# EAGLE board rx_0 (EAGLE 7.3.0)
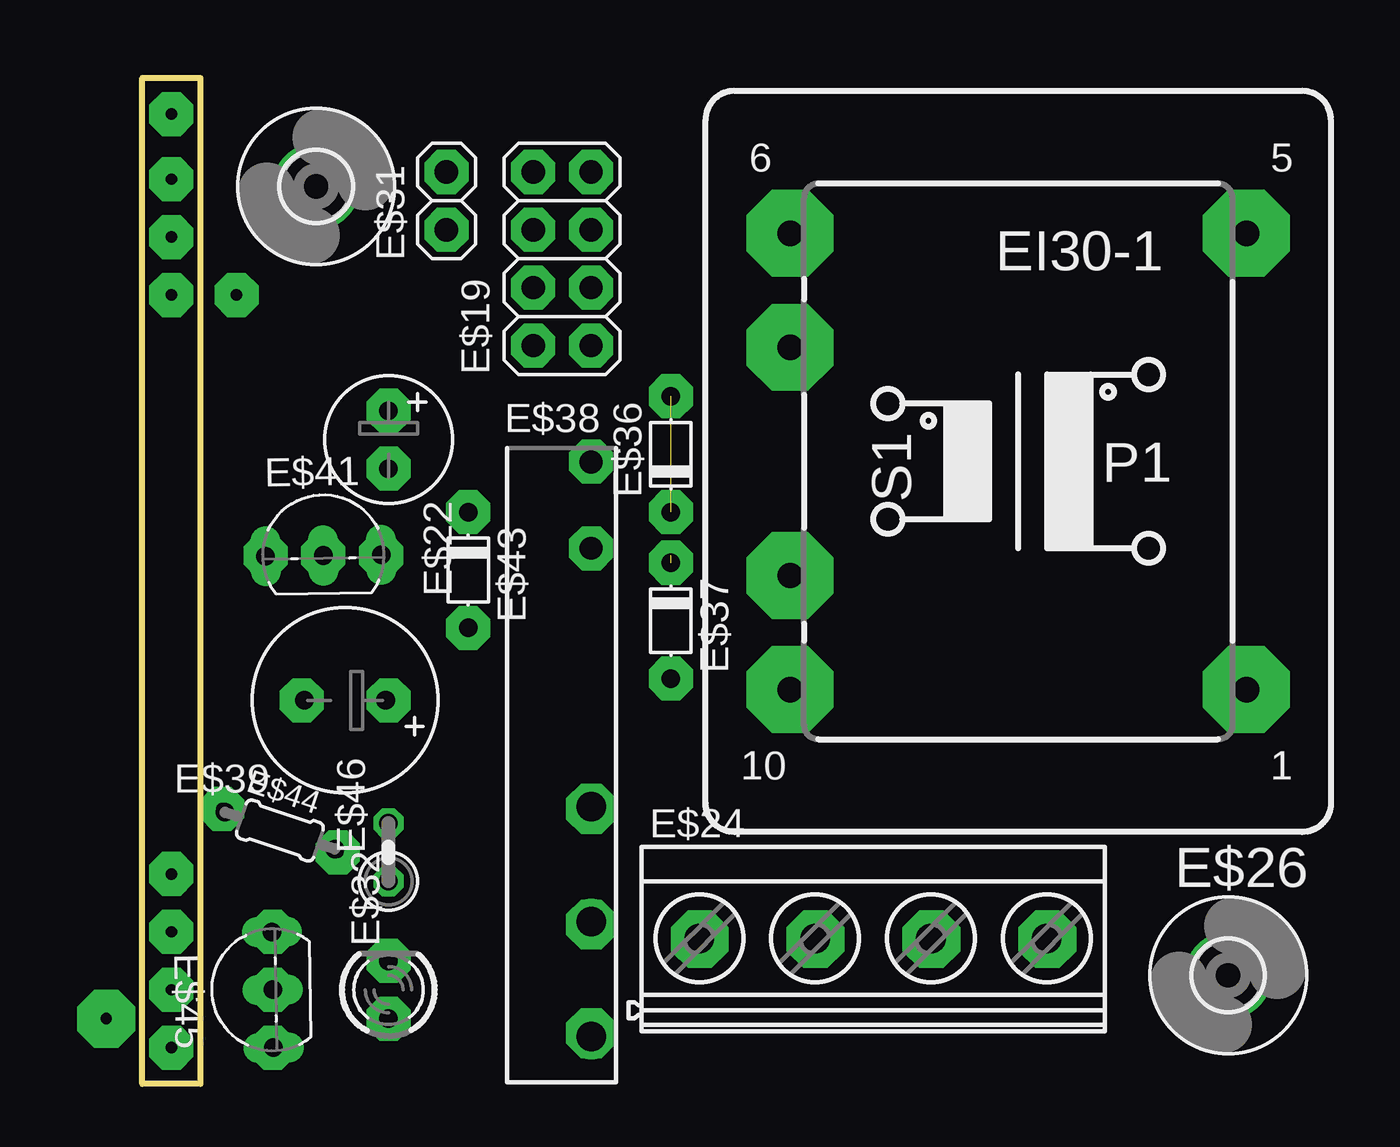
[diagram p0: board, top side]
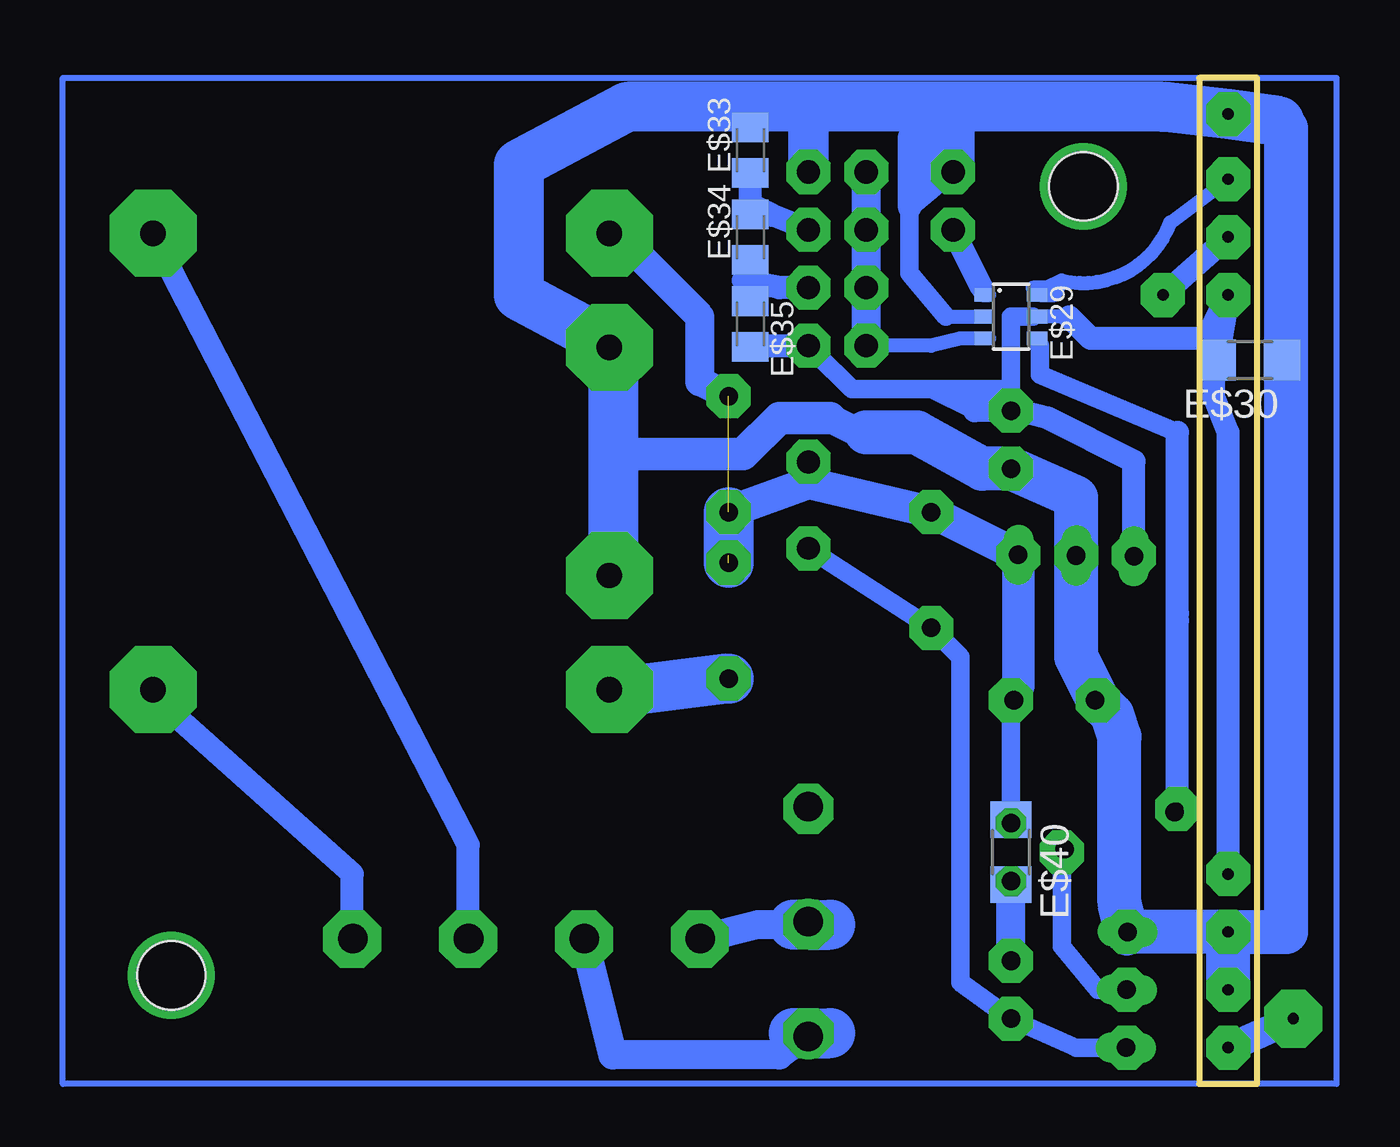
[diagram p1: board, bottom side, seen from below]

Size 2.54 x 44.13 mm. Coordinates in mm from the lower left corner, seen from the top.
Outline: 0,44.13 2.54,44.13 2.54,0 0,0 0,44.13
Copper layers (1*16): Top 0.035mm / dielectric 1.5mm / Bottom 0.035mm
Design rules "default": minimum track width 10mil, minimum drill 24mil, track to track 8mil, track to pad 8mil, pad to pad 8mil, via to via 8mil, smd to smd 8mil, copper to edge 40mil, drill to drill 8mil, minimum pad ring 10mil, minimum via ring 8mil, stop-mask expansion 4mil, vias tented up to drill 0mil, thermal gap 10mil

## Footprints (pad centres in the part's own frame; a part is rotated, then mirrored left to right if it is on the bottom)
2X04 = drill 1.016 octagon: 1 -3.81,-1.27; 2 -3.81,1.27; 3 -1.27,-1.27; 4 -1.27,1.27; 5 1.27,-1.27; 6 1.27,1.27; 7 3.81,-1.27; 8 3.81,1.27
E2,5-6 = drill 0.813 pad 1.6: + -1.27,0 | drill 0.813 pad 1.6 octagon: - 1.27,0
MKDSN1,5/4-5,08 = drill 1.3 pad 2: 1 -7.641,0.025; 2 -2.561,0.025; 3 2.519,0.025; 4 7.599,0.025
EI30-1 = drill 1.118 pad 3.81 octagon: 1 -10.008,10.008; 5 -10.008,-10.008; 6 10.008,-10.008; 7 10.008,-5.004; 9 10.008,5.004; 10 10.008,10.008
3,0 = hole 3: 0,0
SOT23-6 = smd 0.6 x 0.9: 1 -0.95,-1.15; 2 0,-1.15; 3 0.95,-1.15; 4 0.95,1.15; 5 0,1.15; 6 -0.95,1.15
R1206 = smd 1.6 x 1.803: 1 -1.422,0; 2 1.422,0
1X02 = drill 1.016 octagon: 1 -1.27,0; 2 1.27,0
LED3MM = drill 0.813 octagon: A -1.27,0; K 1.27,0
C0805K = smd 1.3 x 1.6: 1 -1,0; 2 1,0
D-5 = drill 0.813 octagon: A 2.54,0; C -2.54,0
FTR-LYC = drill 1 pad 1.6: 1 -3.78,0; 2 0,0 | drill 1.3 pad 2: 3 11.34,0; 4 16.38,0; 5 21.42,0
E3,5-8 = drill 0.813 pad 1.6: + -1.778,0 | drill 0.813 pad 1.6 octagon: - 1.778,0
TO92-BCE = drill 0.813 long: B 2.54,0; C 0,0; E -2.54,0
0204/5 = drill 0.813 octagon: 1 -2.54,0; 2 2.54,0
0207/2V = drill 0.813 octagon: 1 -1.27,0; 2 1.27,0

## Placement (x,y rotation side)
E$19  [2X04]  18.41,36.2 90 top  (outside the outline)
E$22  [E2,5-6]  not placed on the board
E$24  [MKDSN1,5/4-5,08]  not placed on the board
E$26  [EI30-1]  not placed on the board
E$28  [3,0]  not placed on the board
E$29  [SOT23-6]  not placed on the board
E$30  [R1206]  0.32,31.75 180 bottom
E$31  [1X02]  not placed on the board
E$32  [LED3MM]  10.8,4.13 90 top  (outside the outline)
E$33  [C0805K]  not placed on the board
E$34  [C0805K]  not placed on the board
E$35  [C0805K]  not placed on the board
E$36  [D-5]  not placed on the board
E$37  [D-5]  not placed on the board
E$38  [FTR-LYC]  not placed on the board
E$39  [E3,5-8]  not placed on the board
E$40  [R1206]  not placed on the board
E$41  [TO92-BCE]  7.94,23.18 0.9 top
E$42  [3,0]  not placed on the board
E$43  [D-5]  not placed on the board
E$44  [0204/5]  6.03,11.11 341.5 top
E$45  [TO92-BCE]  not placed on the board
E$46  [0207/2V]  10.8,10.16 90 top  (outside the outline)

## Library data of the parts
E$19 = pinhead
E$22 E$30 E$33-E$35 E$39 E$40 E$44 E$46 = rcl
E$24 = con-phoenix-508
E$26 = trafo
E$28 E$42 = holes
E$29 = microchip
E$31 = pinhead_hex
E$32 = led
E$36 E$37 E$43 = diode
E$38 = relay
E$41 E$45 = transistor-npn

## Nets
S$44: E$19.5
S$45: E$19.3
S$61: E$19.2
S$84: E$19.7
S$97: E$32.A
S$109: E$46.1

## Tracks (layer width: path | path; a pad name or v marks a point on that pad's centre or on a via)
S$39  (via drill 0.5 pad 1.93)
  Bottom 1.016: v1.27,37.15 v4.13,34.61
S$43  (via drill 0.5 pad 1.93, 0.5 pad 2.54)
  Bottom 1.27: v-1.59,2.86 v1.27,1.59
S$44
  Bottom 1.016: E$19.5 21.27,38.1 21.91,38.42 22.23,38.42 22.23,39.69
S$45
  Bottom 1.016: E$19.3 20.95,34.92 22.54,35.24
S$46
  Bottom 0.254: 52.39,0 52.39,44.13 -3.49,44.13 -3.49,0 52.39,0
S$47  (via drill 0.5 pad 1.93)
  other vias: 19.69,40.01
S$49  (via drill 0.5 pad 1.93)
  other vias: 17.15,34.92
S$52  (via drill 0.5 pad 1.93)
  other vias: 19.69,37.46
S$54  (via drill 0.5 pad 1.93)
  other vias: 19.69,34.92
S$55  (via drill 0.5 pad 1.93)
  other vias: 17.15,37.46
S$56  (via drill 0.5 pad 1.93)
  other vias: 17.15,32.38
S$57  (via drill 0.5 pad 1.93)  (2 unrouted)
  Bottom 1.27: 28.26,37.46 24.45,33.66 24.45,30.8 v23.18,30.16 | 23.18,23.18 v23.18,25.08
  other vias: 23.18,22.86
S$58  (via drill 0.5 pad 2.54)
  Bottom 1.016: v48.58,17.14 39.69,9.21 v39.69,6.35
S$59  (via drill 0.5 pad 2.54)
  Bottom 1.016: v34.61,6.35 34.61,10.48 v48.58,37.46
S$60  (via drill 0.5 pad 1.93)
  Bottom 2.184: v23.18,17.78 28.26,17.14
S$61  (via drill 0.5 pad 1.93)
  Bottom 1.27: E$19.2 v17.15,40.01
S$63  (via drill 0.6 pad 3.81)
  other vias: 47.62,4.76
S$64
  Bottom 1.93: 13.34,40.01 13.34,42.23
S$65  (via drill 0.6 pad 3.81)
  other vias: 7.62,39.37
S$66
  Bottom 0.61: 11.75,32.7 13.02,32.7 14.29,32.38 17.15,32.38
S$67  (via drill 0.5 pad 1.93)
  Bottom 0.61: 13.65,33.66 12.07,33.66
  Bottom 0.813: v13.34,40.01 15.24,38.42 15.24,35.56 13.65,33.66
  Bottom 1.016: 15.24,38.42 15.24,41.59
S$71
  Bottom 1.016: 3.49,12.07 3.49,20.64
S$74
  Bottom 0.813: 9.53,32.38 9.53,31.11 3.49,28.57
  Bottom 1.016: 3.49,20.32 3.49,28.57
S$75  (via drill 0.5 pad 2.54)
  other vias: 28.26,37.46
S$76  (via drill 0.5 pad 2.54)
  other vias: 28.26,32.07
S$77  (via drill 0.5 pad 2.54)
  other vias: 28.26,22.22
S$78  (via drill 0.5 pad 2.54)
  other vias: 28.26,17.14
S$79  (via drill 0.5 pad 2.18, 0.5 pad 2.54)
  Bottom 1.27: 20.32,6.99 21.91,6.99 v24.45,6.35
  Bottom 2.184: 18.73,6.99 v19.69,6.99 20.32,6.99
S$80  (via drill 0.5 pad 2.18, 0.5 pad 2.54)
  Bottom 1.27: v19.69,2.22 20.95,1.27 28.26,1.27 v29.53,6.35
  Bottom 2.184: v19.69,2.22 18.73,2.22
S$81  (via drill 0.5 pad 2.18)
  other vias: 19.69,12.07
S$82  (via drill 0.5 pad 1.93)
  Bottom 0.813: 19.37,32.07 17.78,30.48 14.29,30.48 | 9.84,33.66 10.8,33.66 10.8,30.48 | 12.38,29.53 14.29,30.48 | v10.8,29.53 10.8,30.48 | 14.29,30.48 10.8,30.48
  Bottom 1.016: 19.37,32.07 v19.69,32.38 22.23,32.38 | 12.38,29.53 v10.8,29.53 10.48,29.53 9.21,29.21 5.4,27.3 v5.4,23.18
S$84  (via drill 0.5 pad 1.93)
  Bottom 1.778: 19.69,42.86 E$19.7 | -1.27,41.91 -0.95,42.23
  Bottom 1.93: -1.27,21.91 -1.27,41.91
  Bottom 2.184: 28.26,22.22 28.26,32.38 32.39,34.61 32.39,40.32 27.62,42.86 19.69,42.86 4.13,42.86 v1.27,42.55 -0.95,42.23
S$86  (via drill 0.5 pad 1.93)
  Bottom 1.016: v1.27,9.21 1.27,21.59
S$87  (via drill 0.5 pad 1.93)
  Bottom 0.406: v1.27,34.61 1.27,34.92
  Bottom 0.61: 7.3,32.7 8.57,33.66 9.53,33.66
  Bottom 1.016: 1.27,21.27 1.27,28.57 1.91,30.16 1.91,33.34 v1.27,34.61 1.59,32.7 7.3,32.7 8.26,33.66
S$88  (via drill 0.5 pad 1.93)
  other vias: 14.29,20
S$89  (via drill 0.5 pad 1.93)
  other vias: 10.8,2.86
S$90  (via drill 0.5 pad 1.93)
  Bottom 1.27: v19.69,27.3 19.69,26.67
S$91
  Bottom 0.61: 12.07,34.61 11.75,34.61
S$92  (via drill 0.5 pad 1.93)
  Bottom 1.016: 12.07,34.92 v13.34,37.46
S$93
  Bottom 1.016: 14.61,41.91 14.61,39.69
S$94  (via drill 0.5 pad 1.93)
  Bottom 0.61: 9.53,34.61 8.89,34.61 8.57,35.24 | 8.57,35.24 arc-83 3.81,37.78 v1.27,39.69 | 8.57,35.24 9.21,34.92 9.84,34.92
S$95
  Bottom 0.813: 5.72,4.13 6.99,4.13 8.57,6.03 8.57,10.16
S$96  (via drill 0.5 pad 1.93)
  Bottom 0.813: 10.8,11.43 v10.8,16.83
  Bottom 1.422: 23.18,25.08 19.69,26.35 v14.29,25.08 v10.48,23.18 10.48,17.46 v10.8,16.83
  Bottom 2.184: 23.18,25.08 23.18,22.86
S$97  (via drill 0.5 pad 1.93)
  Bottom 0.813: v19.69,23.49 14.29,20 13.02,18.73 13.02,4.45 E$32.A
S$98
  Bottom 0.813: 10.8,2.86 7.94,1.59 5.4,1.59
S$99  (via drill 0.5 pad 1.93)
  other vias: 3.49,12.07
S$100  (via drill 0.5 pad 1.93)
  other vias: 8.57,10.16
S$101  (via drill 0.5 pad 1.93)
  other vias: 5.72,4.13
S$102  (via drill 0.5 pad 1.93)
  other vias: 5.72,1.59
S$103
  Bottom 1.422: 5.72,6.35 6.03,7.3
S$104  (via drill 0.5 pad 1.93)
  Bottom 1.93: -1.27,22.22 -1.27,6.67 v1.27,6.67 | v1.27,6.67 v5.72,6.67 6.03,7.94 6.03,15.24 6.35,16.19 v6.99,16.83 7.94,18.73 v7.94,23.18 7.94,25.72 v10.8,26.99 12.07,26.99 14.92,28.57 17.15,28.57 | v1.27,4.13 v1.27,6.67
S$106
  Bottom 1.27: 18.73,29.21 17.46,28.57
  Bottom 1.422: 28.26,29.21 28.26,27.62 22.54,27.62 20.95,29.21 18.73,29.21
S$107
  Bottom 1.27: 11.11,30.16 12.07,30.16
S$108
  Bottom 2.184: 20,2.22 20.32,2.22
S$109  (via drill 0.5 pad 1.93)
  Bottom 1.27: v10.8,5.4 E$46.1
